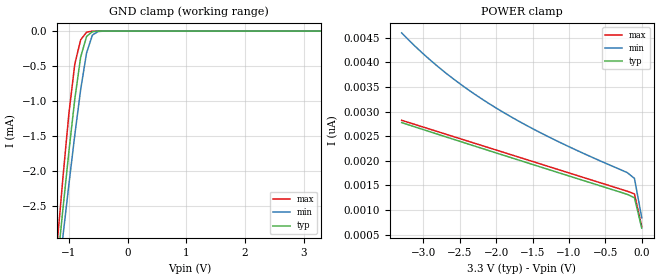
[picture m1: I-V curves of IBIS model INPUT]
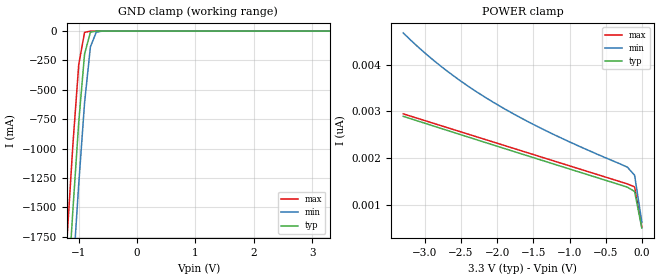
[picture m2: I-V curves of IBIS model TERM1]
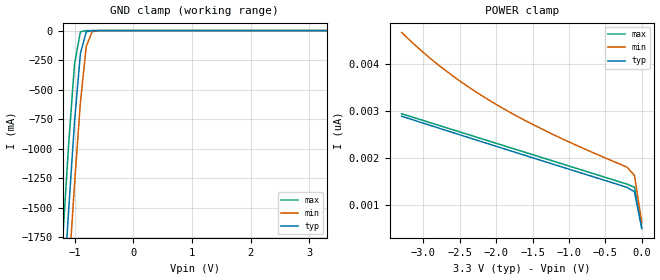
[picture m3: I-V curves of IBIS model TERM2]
|   PERICOM SEMICONDUCTOR CORP
|   IBIS Model of PI3CH480
|   Product Family: 3CH
|   TSSOP (L) Package
[IBIS Ver] 3.2
[Comment char] |_char
[File Name] pi3ch480_l_33v.ibs
[File Rev] 1.0
[Source] File originated at Pericom Semiconductor Corp.
[Date] 11/20/15
[Disclaimer] (C) Copyright PERICOM Semiconductor Corporation
   All rights reserved
  Pericom Semiconductor Corporation hereby grants the user of
  this IBIS model a non-exclusive, nontransferable license to
  use this IBIS model under the following terms.
  This IBIS model is provided on an "AS IS" basis and Pericom
  makes absolutely no warranty with respect to the information
  contained herein. PERICOM DISCLAIMS AND CUSTOMER WAIVES ALL
  WARRANTIES, EXPRESSED OR IMPLIED, INCLUDING WARRANTIES OF
  MERCHANTABILITY OR FITNESS FOR A PARTICULAR PURPOSE. The
  entire risk as to quality and performance is with the customer.
  Accordingly, in no event shall the company be liable for any
  damages, whether in contract or tort, including any lost
  profits or other incidental, consequential, exemplary, or
  punitive damages arising out of the use or application of the
  IBIS model provided in this package. Further, Pericom reserves
  the right to make changes without notice to any product herein
  to improve reliability, function, or design. Pericom does not
  convey any license under patent rights or any other intellectual
  property rights, including those of third parties.
  The user is granted this license only to use the IBIS model
  and is not granted rights to sell, load, rent, lease or license
  the IBIS model in whole or in part, or in modified form to anyone
  other than user. User may modify the IBIS model to suit its specific
  application but rights to derivative works and such modifications
  shall belong to Pericom.
  Pericom is not obligated to provide maintenance or support
  for the licensed IBIS model.
  Contact Pericom at ATTN: APPLICATION ENGINEERING / IBIS MODELS
  1545 Barber Lane Milpitas, CA 95035 USA.
[Component] PI3CH480
[Manufacturer] Pericom Semiconductor Corp.
[Package]
| variable   typ   min   max
R_pkg   0.05122ohm   0.05070ohm   0.05174ohm
L_pkg   2.82616nH   2.45517nH   3.19714nH
C_pkg   0.42513pF   0.33872pF   0.51154pF
[Pin]   signal_name   model_name   R_pin   L_pin   C_pin
1   S   INPUT   0.05174   3.19714nH   0.51154pF
2   IA0   TERM1   0.05140   2.94981nH   0.45394pF
3   IA1   TERM1   0.05105   2.70250nH   0.39633pF
4   YA   TERM2   0.05070   2.45517nH   0.33872pF
5   IB0   TERM1   0.05070   2.45517nH   0.33872pF
6   IB1   TERM1   0.05105   2.70250nH   0.39633pF
7   YB   TERM2   0.05140   2.94981nH   0.45394pF
8   GND   GND   0.05174   3.19714nH   0.51154pF
9   YC   TERM2   0.05174   3.19714nH   0.51154pF
10   IC1   TERM1   0.05140   2.94981nH   0.45394pF
11   IC0   TERM1   0.05105   2.70250nH   0.39633pF
12   YD   TERM2   0.05070   2.45517nH   0.33872pF
13   ID1   TERM1   0.05070   2.45517nH   0.33872pF
14   ID0   TERM1   0.05105   2.70250nH   0.39633pF
15   _EN   INPUT   0.05140   2.94981nH   0.45394pF
16   VCC   POWER   0.05174   3.19714nH   0.51154pF
[Series Switch Groups]
On 1 /
Off 2 /
[Series Pin Mapping]   pin_2   model_name  function_table_group
2   4   SWITCH1   1
5   7   SWITCH1   1
11   9   SWITCH1   1
14   12   SWITCH1   1
3   4   SWITCH1   2
6   7   SWITCH1   2
10   9   SWITCH1   2
13   12   SWITCH1   2
|   Model SWITCH1
[Model] SWITCH1
Model_type Series_switch
| variable   typ   min   max
C_comp   6.40pF   6.30pF   6.50pF
[Voltage Range]   3.300V   2.970V   3.630V
[GND Clamp Reference]   0.000V   0.000V   0.000V
[POWER Clamp Reference]   3.300V   2.970V   3.630V
[On]
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[OFF]
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| Models and submodels in the file (4): INPUT (Input), SWITCH1 (Series_switch), TERM1 (Terminator), TERM2 (Terminator)
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|   Model INPUT
[Model] INPUT
Model_type Input
Vinl = 0.800V
Vinh = 2.000V
| variable   typ   min   max
C_comp   1.800pF   1.700pF   1.900pF
[Voltage Range]   3.300V   2.970V   3.630V
[GND Clamp Reference]   0.000V   0.000V   0.000V
[POWER Clamp Reference]   3.300V   2.970V   3.630V
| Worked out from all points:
|   GND clamp passes 1 mA (typ) near -0.90 V on its own axis
[GND Clamp]
| Voltage   I(typ)   I(min)   I(max)
-3.3V     -21.68mA   -19.86mA   -24.66mA
-1.2V     -3.364mA   -3.668mA   -3.042mA
-1.1V     -2.528mA   -2.921mA   -2.075mA
-1V       -1.72mA    -2.189mA   -1.175mA
-900mV    -970.6uA   -1.485mA   -470.9uA
-800mV    -370.2uA   -835.9uA   -124.8uA
-700mV    -77.27uA   -313.6uA   -15.69uA
-600mV    -8.132uA   -56.97uA   -899.1nA
-500mV    -581.9nA   -5.514uA   -27.41nA
3.3V      630.8pA    1.843nA    27.48pA
[POWER Clamp]   |Note: Vtable = Vcc - Voutput
| Voltage   I(typ)   I(min)   I(max)
-3.3V     2.775nA    4.597nA    2.822nA
-3V       2.631nA    4.167nA    2.682nA
-2.7V     2.489nA    3.79nA     2.543nA
-2.4V     2.347nA    3.458nA    2.403nA
-2V       2.159nA    3.07nA     2.217nA
-1.6V     1.971nA    2.731nA    2.031nA
-1.2V     1.784nA    2.427nA    1.845nA
-800mV    1.597nA    2.149nA    1.66nA
-200mV    1.318nA    1.76nA     1.381nA
-100mV    1.248nA    1.64nA     1.327nA
0V        630.8pA    841.6pA    663.1pA
|   Model TERM1
[Model] TERM1
Model_type Terminator
| variable   typ   min   max
C_comp   3.200pF   3.150pF   3.350pF
[Voltage Range]   3.300V   2.970V   3.630V
[GND Clamp Reference]   0.000V   0.000V   0.000V
[POWER Clamp Reference]   3.300V   2.970V   3.630V
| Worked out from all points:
|   GND clamp passes 1 mA (typ) near -0.71 V on its own axis
[GND Clamp]
| Voltage   I(typ)   I(min)   I(max)
-3.3V     -18.92A    -19.03A    -18.85A
-1.2V     -2.312A    -2.839A    -1.76A
-1.1V     -1.522A    -2.068A    -964.6mA
-1V       -774.2mA   -1.302A    -284.3mA
-900mV    -194.8mA   -609.8mA   -10.78mA
-800mV    -10.29mA   -134.3mA   -175.3uA
-700mV    -368.5uA   -9.267mA   -1.643uA
-500mV    -243.7nA   -27.78uA   -136.6pA
3.3V      494.6pA    1.892nA    95.6pA
[POWER Clamp]   |Note: Vtable = Vcc - Voutput
| Voltage   I(typ)   I(min)   I(max)
-3.3V     2.893nA    4.681nA    2.946nA
-3V       2.744nA    4.25nA     2.8nA
-2.7V     2.595nA    3.872nA    2.655nA
-2.4V     2.447nA    3.537nA    2.509nA
-2V       2.251nA    3.144nA    2.315nA
-1.6V     2.056nA    2.799nA    2.121nA
-1.2V     1.861nA    2.49nA     1.928nA
-200mV    1.374nA    1.803nA    1.443nA
-100mV    1.281nA    1.63nA     1.379nA
0V        494.6pA    626.1pA    523.5pA
|   Model TERM2
[Model] TERM2
Model_type Terminator
| variable   typ   min   max
C_comp   3.200pF   3.150pF   3.350pF
[Voltage Range]   3.300V   2.970V   3.630V
[GND Clamp Reference]   0.000V   0.000V   0.000V
[POWER Clamp Reference]   3.300V   2.970V   3.630V
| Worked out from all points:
|   GND clamp passes 1 mA (typ) near -0.71 V on its own axis
[GND Clamp]
| Voltage   I(typ)   I(min)   I(max)
-3.3V     -18.92A    -19.03A    -18.85A
-1.2V     -2.312A    -2.839A    -1.76A
-1.1V     -1.522A    -2.068A    -964.6mA
-1V       -774.2mA   -1.302A    -284.3mA
-900mV    -194.8mA   -609.8mA   -10.79mA
-800mV    -10.29mA   -134.3mA   -176uA
-700mV    -369.5uA   -9.267mA   -1.644uA
-500mV    -244.1nA   -27.85uA   -136.6pA
3.3V      494.7pA    1.892nA    95.64pA
[POWER Clamp]   |Note: Vtable = Vcc - Voutput
| Voltage   I(typ)   I(min)   I(max)
-3.3V     2.893nA    4.681nA    2.946nA
-3V       2.744nA    4.25nA     2.8nA
-2.7V     2.595nA    3.872nA    2.655nA
-2.4V     2.448nA    3.537nA    2.509nA
-2V       2.251nA    3.144nA    2.315nA
-1.6V     2.056nA    2.799nA    2.122nA
-1.2V     1.861nA    2.49nA     1.928nA
-200mV    1.374nA    1.803nA    1.444nA
-100mV    1.281nA    1.63nA     1.379nA
0V        494.7pA    626.1pA    523.5pA
